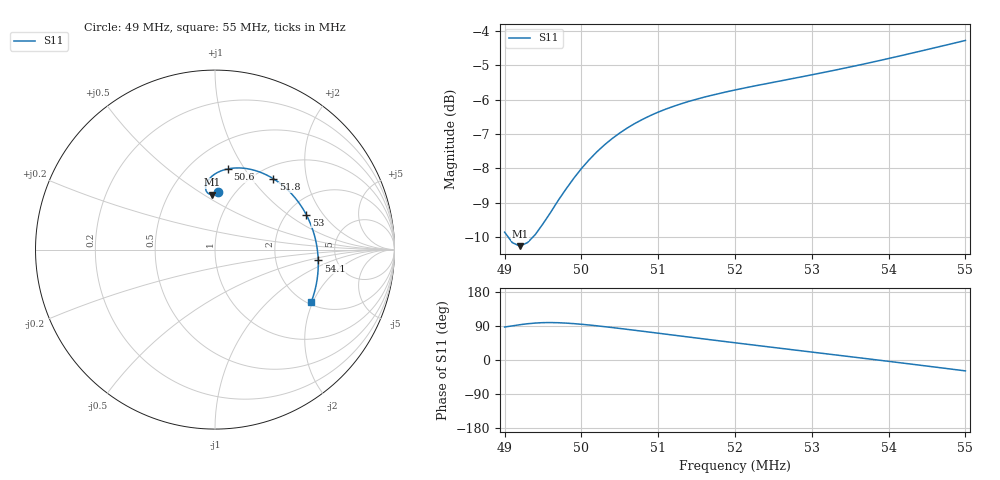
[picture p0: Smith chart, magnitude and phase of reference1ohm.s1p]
# MHz S RI R 1
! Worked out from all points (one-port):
!   61 points, 49 MHz to 55 MHz, reference 1 ohm
!   lowest |S11| = -10.3 dB at 49.2 MHz (marker M1), VSWR 1.88, Z = 0.803 + j0.543 ohm
!   |S11| at or under -10 dB: 49.05 MHz to 49.37 MHz (322.2 kHz wide, 0.655 % of centre)
!   S11 on the Smith chart (normalised r, x): 49 MHz: 0.84, +0.60; 50.6 MHz: 0.75, +0.85; 51.8 MHz: 1.21, +1.29; 53 MHz: 2.52, +1.39; 54.1 MHz: 3.61, -0.66; 55 MHz: 2.08, -1.95
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49  0.0169 0.321
49.1  -0.000113 0.3103
49.2  -0.0168 0.3062
49.3  -0.0309 0.3089
49.5  -0.0493 0.3269
49.7  -0.052 0.3539
49.8  -0.0475 0.3684
49.9  -0.04 0.3828
50.1  -0.0168 0.4091
50.3  0.0151 0.4302
50.5  0.0526 0.445
50.6  0.0729 0.4499
50.9  0.1369 0.4549
51.1  0.1805 0.4506
51.3  0.2237 0.4406
51.6  0.2862 0.4163
51.8  0.3256 0.3945
52  0.3628 0.369
52.4  0.4296 0.3075
52.8  0.4852 0.2347
53  0.5085 0.1946
53.3  0.5374 0.1303
53.5  0.5525 0.085
53.8  0.5682 0.0138
54.1  0.5752 -0.0607
54.3  0.5746 -0.1117
54.7  0.5596 -0.2156
55  0.5356 -0.2936
